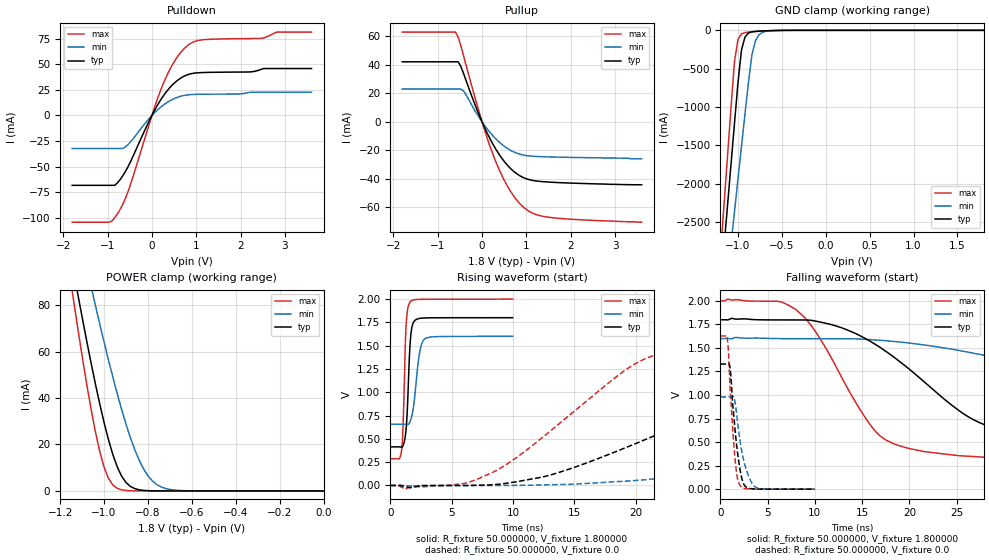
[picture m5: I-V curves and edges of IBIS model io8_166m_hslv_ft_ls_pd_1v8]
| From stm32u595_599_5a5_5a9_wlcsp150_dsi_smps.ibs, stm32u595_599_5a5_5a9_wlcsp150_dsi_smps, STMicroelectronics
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|   Model io8_166m_hslv_ft_ls_pd_1v8
[Model]  io8_166m_hslv_ft_ls_pd_1v8
Model_type I/O
Polarity   Non-Inverting
Enable   Active-Low
Vinl =   0.540000V
Vinh =   1.260000V
Vmeas =  0.900000V
Cref =   50.000000pF
Rref =   100.000000M
Vref =   0.0V
C_comp   3.358300pF   3.352700pF   3.400300pF
[Temperature Range]   25.000000   0.140000k   -40.000000
[Pullup Reference]   1.800000V   1.600000V   2.000000V
[Pulldown Reference]   0.0V   0.0V   0.0V
[POWER Clamp Reference]   1.800000V   1.600000V   2.000000V
[GND Clamp Reference]   0.0V   0.0V   0.0V
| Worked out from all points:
|   slope of the pulldown table from 0 to 0.27 V, typ, clamps not added: 13.6 ohm
|   slope of the pullup table from 0 to 0.27 V, typ, clamps not added: 15.9 ohm
|   GND clamp passes 1 mA (typ) near -0.50 V on its own axis
|   POWER clamp passes 1 mA (typ) near -0.86 V on its own axis
|   rising waveform, R_fixture 50.000000, V_fixture 1.800000: 20-80 % time 278ps typ, 481ps min, 228ps max; typ from 0.414 V to 1.8 V
|   rising waveform, R_fixture 50.000000, V_fixture 0.0: 20-80 % time 16.1ns typ, 33.4ns min, 9.36ns max; typ from 0 V to 1.33 V
|   falling waveform, R_fixture 50.000000, V_fixture 1.800000: 20-80 % time 11.2ns typ, 27.7ns min, 6.11ns max; typ from 1.8 V to 0.414 V
|   falling waveform, R_fixture 50.000000, V_fixture 0.0: 20-80 % time 786ps typ, 1.05ns min, 620ps max; typ from 1.33 V to 0 V
[Pulldown]
|Voltage   I(typ)   I(min)   I(max)
-1.8V     -68.38mA   -32.32mA   -104.4mA
-960mV    -68.38mA   -32.32mA   -104.4mA
-780mV    -66.08mA   -32.32mA   -96.43mA
-540mV    -50.22mA   -28.51mA   -74.66mA
0V        -10fA      -700fA     0A
240mV     18.04mA    9.599mA    29.42mA
480mV     30.68mA    16.02mA    50.95mA
780mV     39.48mA    19.98mA    67.56mA
1.14V     41.99mA    20.78mA    74.01mA
2.46V     45.09mA    22.69mA    75.45mA
2.82V     45.91mA    22.69mA    81.58mA
3.6V      45.91mA    22.69mA    81.58mA
[Pullup]
|Voltage   I(typ)   I(min)   I(max)
-1.8V     42.16mA    23.02mA    63.04mA
-600mV    42.16mA    23.02mA    63.04mA
-540mV    42.16mA    23.02mA    59.55mA
-420mV    34.21mA    21.81mA    46.75mA
0V        0A         0A         0A
300mV     -18.63mA   -11.6mA    -27.18mA
600mV     -31.41mA   -19.24mA   -46.67mA
780mV     -36.41mA   -22mA      -54.89mA
960mV     -39.54mA   -23.51mA   -60.64mA
1.2V      -41.44mA   -24.28mA   -64.93mA
1.56V     -42.42mA   -24.69mA   -67.24mA
3.6V      -44.2mA    -26mA      -70.5mA
[GND_clamp]
|Voltage   I(typ)   I(min)   I(max)
-1.8V     -9.908A    -9.683A    -9.994A
-1.2V     -3.383A    -4.084A    -2.934A
-1.16V    -2.841A    -3.655A    -2.294A
-1.12V    -2.299A    -3.226A    -1.656A
-1.04V    -1.218A    -2.369A    -414.2mA
-1V       -684.7mA   -1.941A    -119.2mA
-960mV    -257.2mA   -1.514A    -45.67mA
-920mV    -87.04mA   -1.089A    -28.94mA
-840mV    -19.36mA   -312.8mA   -18.98mA
-800mV    -13.56mA   -132.4mA   -15.51mA
-720mV    -8.053mA   -25.67mA   -9.505mA
1.8V      45.71uA    33.32uA    56.11uA
[POWER_clamp]
|Voltage   I(typ)   I(min)   I(max)
-1.8V     470.8mA    433.7mA    554.6mA
-1.14V    95.25mA    122.7mA    82.82mA
-1.12V    84.97mA    114mA      70.27mA
-1.06V    55.51mA    88.42mA    35.67mA
-1.04V    46.34mA    80.15mA    25.76mA
-1V       29.51mA    64.13mA    10.3mA
-940mV    10.39mA    41.86mA    1.109mA
-900mV    3.624mA    28.77mA    182.8uA
-840mV    490.7uA    13.24mA    11.35uA
-800mV    116.8uA    6.532mA    1.77uA
-740mV    13.2uA     1.724mA    109.3nA
0V        0A         18.75nA    0A
[Ramp]
| variable   typ   min   max
dV/dt_r  0.79740/16.06955n   0.58771/33.32156n   0.97632/9.34819n
dV/dt_f  0.83143/11.14563n   0.56520/27.65093n   1.02745/6.09635n
R_load = 50.000000
[Rising Waveform]
R_fixture= 50.000000
V_fixture= 1.800000
V_fixture_min= 1.600000
V_fixture_max= 2.000000
|time   V(typ)   V(min)   V(max)
0s        413.8mV    656.5mV    287.1mV
920.9ps   410.8mV    656.5mV    378.3mV
1.041ns   428mV      656.5mV    634.6mV
1.221ns   525.3mV    656mV      1.495V
1.301ns   620.3mV    654.6mV    1.741V
1.622ns   1.531V     687.2mV    1.969V
1.922ns   1.755V     872.5mV    1.991V
2.382ns   1.792V     1.418V     1.996V
2.783ns   1.797V     1.57V      1.997V
9.97ns    1.8V       1.599V     2V
[Rising Waveform]
R_fixture= 50.000000
V_fixture= 0.0
V_fixture_min= 0.0
V_fixture_max= 0.0
|time   V(typ)   V(min)   V(max)
0s        1.796nV    144.1nV    1.167nV
7.207ns   2.165mV    -375.6uV   72.9mV
12.81ns   103.6mV    6.763mV    558.8mV
20.42ns   472.3mV    57.37mV    1.338V
28.83ns   913.9mV    198mV      1.556V
35.24ns   1.138V     327mV      1.597V
45.25ns   1.258V     526.2mV    1.619V
62.86ns   1.313V     792.4mV    1.626V
81.28ns   1.326V     910.3mV    1.627V
199.4ns   1.329V     979.7mV    1.627V
[Falling Waveform]
R_fixture= 50.000000
V_fixture= 1.800000
V_fixture_min= 1.600000
V_fixture_max= 2.000000
|time   V(typ)   V(min)   V(max)
0s        1.8V       1.599V     2V
8.008ns   1.797V     1.598V     1.907V
10.01ns   1.786V     1.598V     1.682V
16.82ns   1.512V     1.582V     572.9mV
25.23ns   836.1mV    1.474V     355.6mV
28.83ns   654.8mV    1.402V     334mV
34.43ns   548.2mV    1.266V     312.2mV
48.45ns   462.3mV    936.8mV    293.7mV
65.27ns   430.9mV    778.2mV    288.5mV
199.4ns   413.8mV    656.5mV    287.1mV
[Falling Waveform]
R_fixture= 50.000000
V_fixture= 0.0
V_fixture_min= 0.0
V_fixture_max= 0.0
|time   V(typ)   V(min)   V(max)
0s        1.329V     979.7mV    1.627V
740.7ps   1.329V     979.8mV    1.591V
860.9ps   1.334V     979.9mV    1.444V
1.041ns   1.27V      979.8mV    1.05V
1.502ns   687.1mV    950.7mV    375.4mV
1.742ns   445.8mV    773.1mV    152mV
2.062ns   218.6mV    522.8mV    42.39mV
2.563ns   38.19mV    268.5mV    7.185mV
3.724ns   1.468mV    20.48mV    394.8uV
9.97ns    1.796nV    144.1nV    1.167nV
